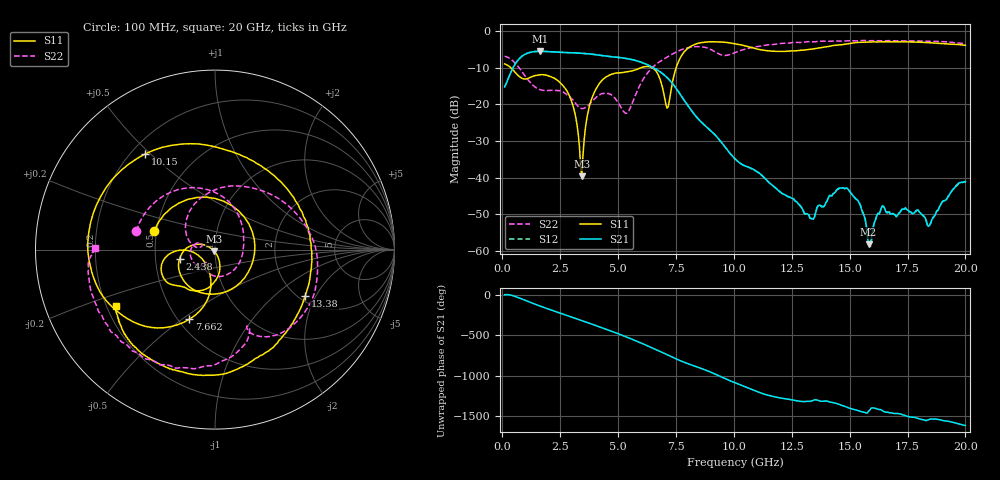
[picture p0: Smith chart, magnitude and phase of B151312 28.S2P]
!  2-Port S-parameters saved by WinCal
! VAR MeasName=S-Parameters (CALIBRATED_DATA) read from VNA (N5244A)
! VAR MeasDate=12/8/2015 5:45:37 PM
! VAR NAME=B151312 28
! VAR FILENAME=B151312 28.S2P
! VAR DATE=12/8/2015 5:45:37 PM
! VAR PHYS_PORTS=1,2
# Hz S DB R 50
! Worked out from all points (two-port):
!   401 points, 100 MHz to 20 GHz, reference 50 ohm
!   highest |S21| = -5.59 dB at 1.642 GHz (marker M1); lowest = -58.2 dB at 15.82 GHz (marker M2)
!   |S21| within 3 dB of the highest: 604.5 MHz to 6.009 GHz (5.405 GHz wide, 163 % of centre)
!   lowest |S11| = -39.6 dB at 3.433 GHz (marker M3), VSWR 1.02, Z = 49.5 - j0.908 ohm
!   |S11| at or under -10 dB: 357.7 MHz to 6.007 GHz (5.649 GHz wide, 178 % of centre); 6.461 GHz to 7.513 GHz (1.051 GHz wide, 15 % of centre)
!   |S22| runs from -22.5 to -2.6 dB; largest |S21 - S12| = 0.0013
!   S11 on the Smith chart (normalised r, x): 100 MHz: 0.49, +0.12; 2.438 GHz: 0.67, -0.07; 7.662 GHz: 0.57, -0.53; 10.15 GHz: 0.25, +0.48; 13.38 GHz: 2.17, -1.64; 20 GHz: 0.24, -0.25
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1e8  -9.02 162.9  -15.27 6.6  -15.27 6.6  -6.92 166.8
8.4625e8  -12.90 15.1  -6.93 -47.1  -6.93 -47.1  -11.07 74.5
1.64225e9  -11.95 -108.4  -5.59 -135.9  -5.59 -135.9  -16.02 1.4
2.43825e9  -13.77 -164.8  -5.84 144.2  -5.84 144.1  -16.27 -75.6
3.03525e9  -20.04 162.5  -5.98 85.4  -5.98 85.4  -18.70 -120.9
3.43325e9  -39.63 -118.5  -6.11 45.2  -6.11 45.2  -21.17 -126.1
3.7815e9  -20.08 -73.9  -6.30 9.4  -6.30 9.5  -19.85 -121.8
4.32875e9  -13.34 -99.9  -6.75 -47.1  -6.75 -47.2  -17.12 -150.8
5.473e9  -11.05 -133.3  -7.66 -172.1  -7.66 -172.2  -21.71 170.1
6.11975e9  -9.79 -146.0  -8.84 109.5  -8.84 109.4  -12.80 134.6
6.7665e9  -12.43 -176.2  -10.96 26.7  -10.97 26.6  -8.54 71.5
7.1645e9  -20.67 -125.9  -13.04 -27.2  -13.02 -27.2  -6.96 40.7
7.662e9  -7.67 -110.1  -17.10 -92.4  -17.06 -92.4  -5.31 7.8
8.80625e9  -3.05 -174.7  -26.09 145.2  -26.08 144.9  -4.59 -52.9
1.005e10  -3.50 130.8  -34.84 -10.0  -34.87 -10.5  -5.94 -67.9
1.01495e10  -3.61 126.3  -35.43 -21.3  -35.47 -21.4  -5.67 -69.1
1.338325e10  -4.97 -27.2  -51.20 125.1  -51.08 124.7  -2.99 -117.6
1.4826e10  -3.63 -73.0  -42.91 53.2  -42.90 53.0  -2.75 -134.5
1.5821e10  -3.03 -97.6  -58.17 -2.1  -58.03 -4.3  -2.69 -144.2
1.67165e10  -3.00 -113.4  -49.52 -23.4  -49.25 -22.6  -2.68 -152.0
1.8408e10  -3.22 -136.9  -53.23 -111.3  -53.12 -111.7  -2.85 -167.1
2e10  -3.94 -150.3  -41.01 178.4  -41.03 176.8  -3.53 179.1
